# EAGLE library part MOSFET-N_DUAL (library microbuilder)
Dual N-Channel MOSFET SOT363 (2.0x1.25mm) 2N7002PS - 60V, 320mA [Digikey: 568-5984-1-ND]
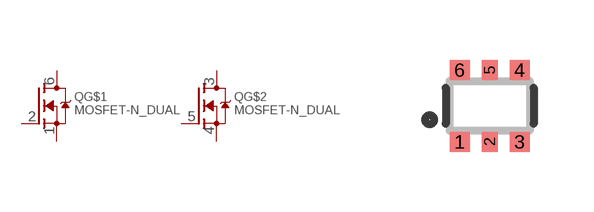
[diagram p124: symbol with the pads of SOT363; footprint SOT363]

Designator prefix Q; gates G$1=MOSFET-N G$2=MOSFET-N

## MOSFET-N_DUAL  [SOT363]
1  G$1:S
2  G$1:G
3  G$2:D
4  G$2:S
5  G$2:G
6  G$1:D

## Footprint SOT363 (pad centres in mm)
Source: http://www.nxp.com/documents/data_sheet/2N7002PS.pdf
smd 0.5 x 0.5: 1 -0.75,-0.9; 3 0.75,-0.9; 4 0.75,0.9; 6 -0.75,0.9
smd 0.4 x 0.5: 2 0,-0.9; 5 0,0.9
